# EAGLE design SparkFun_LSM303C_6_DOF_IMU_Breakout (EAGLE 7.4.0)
DESIGNER: Brent Wilkins; VERSION: v10
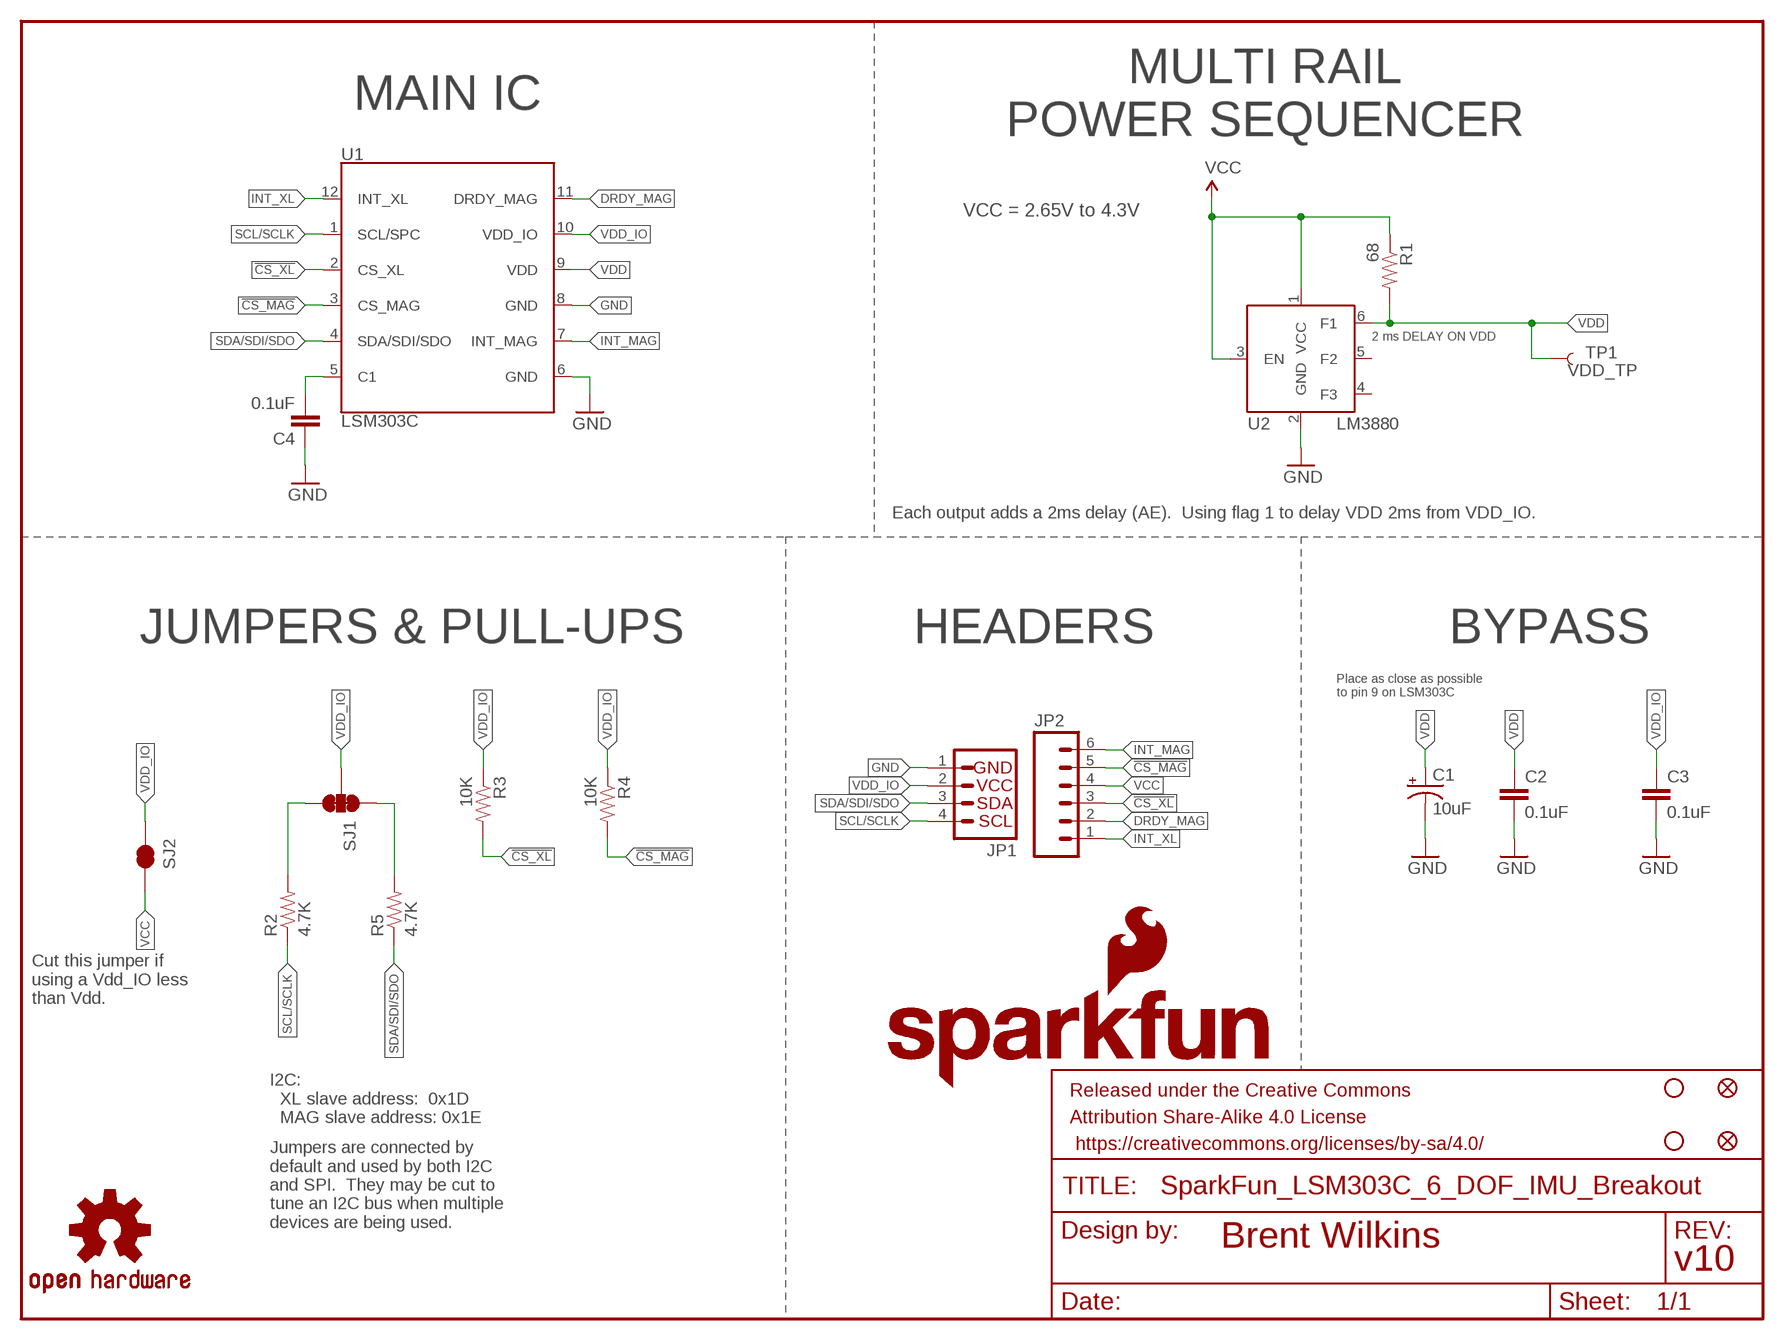
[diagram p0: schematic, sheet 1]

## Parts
C1  10uF  CAP_POL1206  [EIA3216]
C2  0.1uF  0.1UF-25V(+80/-20%)(0603)  [0603-CAP]
C3  0.1uF  0.1UF-25V(+80/-20%)(0603)  [0603-CAP]
C4  0.1uF  0.1UF-25V(+80/-20%)(0603)  [0603-CAP]
FID1  FIDUCIAL1X2  [FIDUCIAL-1X2]
FID2  FIDUCIAL1X2  [FIDUCIAL-1X2]
FRAME1  FRAME-LETTER  [CREATIVE_COMMONS]
JP1  I2C_STANDARD  [1X04]
JP2  M06SILK_FEMALE_PTH  [1X06]
LOGO1  SFE_LOGO_NAME.1_INCH  [SFE_LOGO_NAME_.1]
LOGO2  SFE_LOGO_FLAME.1EXP  [SFE_LOGO_FLAME_COPPER_EXPOSED_.1]
R1  68  RESISTOR0603-RES  [0603-RES]
R2  4.7K  4.7KOHM-1/10W-1%(0603)  [0603-RES]
R3  10K  10KOHM-1/10W-1%(0603)0603  [0603-RES]
R4  10K  10KOHM-1/10W-1%(0603)0603  [0603-RES]
R5  4.7K  4.7KOHM-1/10W-1%(0603)  [0603-RES]
SJ1  JUMPER-PAD-3-NC_BY_TRACE  [PAD-JUMPER-3-3OF3_NC_BY_TRACE_YES_SILK_FULL_BOX]
SJ2  JUMPER-PAD-2-NC_BY_TRACE  [PAD-JUMPER-2-NC_BY_TRACE_YES_SILK]
STANDOFF1  STAND-OFF  [STAND-OFF]
STANDOFF2  STAND-OFF  [STAND-OFF]
TP1  VDD_TP  TEST-POINTTP_15TH_THRU  [TP_15TH]
U1  LSM303C  [LGA-12]
U2  LM3880  LM3880/-QI  [SOT23-6]
U$8  OSHW-LOGOS  [OSHW-LOGO-S]

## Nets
!CS_MAG: JP2.5 R4.2 U1.3(CS_MAG)
!CS_XL: JP2.3 R3.2 U1.2(CS_XL)
DRDY_MAG: JP2.2 U1.11(DRDY_MAG)
GND: C1.C(-) C2.2 C3.2 C4.1 JP1.1 U1.6(GND) U1.8(GND) U2.2(GND)
I2C-UP: R5.2 SJ1.1
INT_MAG: JP2.6 U1.7(INT_MAG)
INT_XL: JP2.1 U1.12(INT_XL)
N$1: C4.2 U1.5(C1)
N$2: R2.2 SJ1.3
SCL/SCLK: JP1.4 R2.1 U1.1(SCL/SPC)
SDA/SDI/SDO: JP1.3 R5.1 U1.4(SDA/SDI/SDO)
VCC: JP2.4 R1.1 SJ2.2 U2.1(VCC) U2.3(EN)
VDD: C1.A(+) C2.1 R1.2 TP1.P$1 U1.9(VDD) U2.6(F1)
VDD_IO: C3.1 JP1.2 R3.1 R4.1 SJ1.2 SJ2.1 U1.10(VDD_IO)
Unconnected: U2.4(F3) U2.5(F2)

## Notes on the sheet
- MAIN IC
- MULTI RAIL
  POWER SEQUENCER
- VCC = 2.65V to 4.3V
- 2 ms DELAY ON VDD
- Each output adds a 2ms delay (AE).  Using flag 1 to delay VDD 2ms from VDD_IO.
- JUMPERS & PULL-UPS | HEADERS | BYPASS
- Place as close as possible
  to pin 9 on LSM303C
- Cut this jumper if
  using a Vdd_IO less
  than Vdd.
- I2C:
    XL slave address:  0x1D
    MAG slave address: 0x1E
- Jumpers are connected by
  default and used by both I2C
  and SPI.  They may be cut to
  tune an I2C bus when multiple
  devices are being used.

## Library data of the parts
C1 = SparkFun:CAP_POL: Capacitor Polarized; PROD_ID: CAP-00811
C2-C4 = SparkFun-Capacitors:0.1UF-25V(+80/-20%)(0603): CAP-00810; PROD_ID: CAP-00810
FID1 FID2 = SparkFun:FIDUCIAL: Fiducial Alignment Points
FRAME1 = SparkFun-Aesthetics:FRAME-LETTER: Schematic Frame
JP1 = SparkFun-Connectors:I2C_STANDARD: SparkFun has standardized on a pinout for all I2C based sensor breakouts. This pinout allows I2C boards to be plugged directly into the headers on Arduino Uno compatible boards, and to be daisy chained easily.
JP2 = SparkFun-Connectors:M06: Header 6 Standard 6-pin 0.1" header. Use with straight break away headers (SKU : PRT-00116), right angle break away headers (PRT-00553), swiss pins (PRT-00743), machine pins (PRT-00117), and female headers (PRT-00115). Molex polarized connector foot print use with SKU : PRT-08094 with associated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; PROD_ID: CONN-08437
LOGO1 = SparkFun-Aesthetics:SFE_LOGO_NAME: SFE Logo, name only
LOGO2 = SparkFun-Aesthetics:SFE_LOGO_FLAME: SFE Logo, flame only
R1 = SparkFun-Passives:RESISTOR: Resistor; PROD_ID: RES-07860
R2 R5 = SparkFun-Resistors:4.7KOHM-1/10W-1%(0603): RES-07857; PROD_ID: RES-07857
R3 R4 = SparkFun-Resistors:10KOHM-1/10W-1%(0603): RES-00824; PROD_ID: RES-00824
SJ1 = SparkFun-Passives:JUMPER-PAD-3-NC_BY_TRACE
SJ2 = SparkFun-Passives:JUMPER-PAD-2-NC_BY_TRACE
STANDOFF1 STANDOFF2 = SparkFun-Electromechanical:STAND-OFF: #4 Stand Off
TP1 = SparkFun-Passives:TEST-POINT: Bare copper test points for troubleshooting or ICT
U1 = SparkFun-DigitalIC:LSM303C: Ultra-compact high-performance eCompass module: 3D accelerometer and 3D magnetometer http://www.st.com/st-web-ui/static/active/en/resource/technical/document/datasheet/DM00089896.pdf; PROD_ID: IC-12557
U2 = SparkFun-DigitalIC:LM3880/-QI: Simple Power Sequencer Precision enable pin & 3 open-drain output flags Input Voltage Range of 2.7 V to 5.5 V Power-Up and Power-Down Control LM3880MF-1XY (Timing Designator) AF16ms AE2ms AA10ms AB30ms AC60ms AD120ms The timing sequence of the LM3880 is controlled entirely by the enable (EN) pin.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; PROD_ID: IC-12558
U$8 = SparkFun:OSHW-LOGO: Open Source Hardware Logo This logo indicates the piece of hardware it is found on incorporates a OSHW license and/or adheres to the definition of open source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

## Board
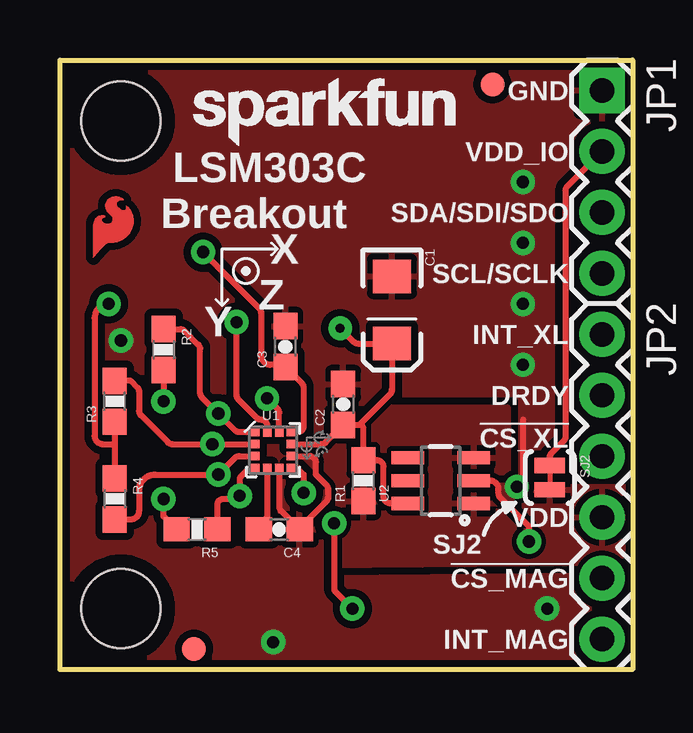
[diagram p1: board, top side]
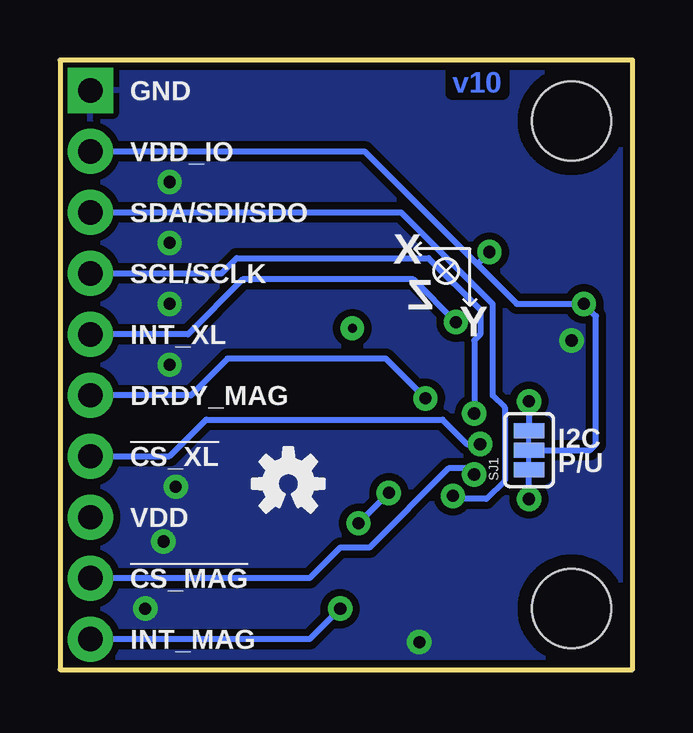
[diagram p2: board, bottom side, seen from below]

Size 23.88 x 25.4 mm. Coordinates in mm from the lower left corner, seen from the top.
Outline: 0,0 0,25.4 23.88,25.4 23.88,0 0,0
Copper layers (1*16): Top 0.035mm / dielectric 1.5mm / Bottom 0.035mm
Design rules "SparkFun-2-layer": minimum track width 7mil, minimum drill 15mil, track to track 8mil, track to pad 8mil, pad to pad 8mil, via to via 8mil, smd to smd 8mil, copper to edge 8mil, drill to drill 8mil, minimum pad ring 12mil, minimum via ring 10mil, stop-mask expansion 4mil, vias tented up to drill 20mil, thermal gap 10mil

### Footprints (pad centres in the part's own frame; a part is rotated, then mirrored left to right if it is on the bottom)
EIA3216 = smd 1.4 x 1.6: A 1.4,0; C -1.4,0
0603-CAP = smd 1.1 x 1: 1 -0.85,0; 2 0.85,0
FIDUCIAL-1X2 = smd 1 x 1: 1 0,0
1X04 = drill 1.016 pad 1.88 square: 1 0,0 | drill 1.016 pad 1.88: 2 2.54,0; 3 5.08,0; 4 7.62,0
1X06 = drill 1.016 pad 1.88: 1 0,0; 2 2.54,0; 3 5.08,0; 4 7.62,0; 5 10.16,0; 6 12.7,0
0603-RES = smd 1.1 x 1: 1 -0.85,0; 2 0.85,0
PAD-JUMPER-3-3OF3_NC_BY_TRACE_YES_SILK_FULL_BOX = smd 0.635 x 1.27: 1 -0.813,0; 2 0,0; 3 0.813,0
PAD-JUMPER-2-NC_BY_TRACE_YES_SILK = smd 0.635 x 1.27: 1 -0.508,0; 2 0.508,0
STAND-OFF = hole 3.302: 0,0
TP_15TH = drill 0.381 pad 0.61: P$1 0,0
LGA-12 = smd 0.375 x 0.35: 1 -0.75,0.75; 2 -0.75,0.25; 3 -0.75,-0.25; 4 -0.75,-0.75; 7 0.75,-0.75; 8 0.75,-0.25; 9 0.75,0.25; 10 0.75,0.75 | smd 0.35 x 0.375: 5 -0.25,-0.75; 6 0.25,-0.75; 11 0.25,0.75; 12 -0.25,0.75
SOT23-6 = smd 0.55 x 1.35: 1 -0.95,-1.375; 2 0,-1.375; 3 0.95,-1.375; 4 0.95,1.375; 5 0,1.375; 6 -0.95,1.375

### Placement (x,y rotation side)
C1  13.84,14.99 270 top
C2  11.81,11.05 90 top
C3  9.4,13.46 90 top
C4  9.14,5.84 180 top
FID1  18.03,24.38 0 top
FID2  5.59,0.86 0 top
FRAME1  not placed on the board
JP1  22.61,24.13 270 top
JP2  22.61,13.97 270 top
LOGO1  5.08,21.34 0 top
LOGO2  1.07,16.81 0 top
R1  12.65,7.87 90 top
R2  4.32,13.34 270 top
R3  2.29,11.18 90 top
R4  2.29,7.11 270 top
R5  5.71,5.84 180 top
SJ1  4.32,9.14 90 bottom
SJ2  20.42,8 270 top
STANDOFF1  2.54,22.86 0 top
STANDOFF2  2.54,2.54 0 top
TP1  11.68,14.22 0 top
U1  8.89,9.14 0 top
U2  15.88,7.87 90 top
U$8  14.35,7.75 0 bottom

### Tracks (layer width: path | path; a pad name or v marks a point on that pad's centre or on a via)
!CS_MAG  (via drill 0.51)
  Top 0.254: U1.3 7.47,8.89 arc45 7.3,8.82 v6.6,8.13 3.98,8.13 arc90 3.3,7.45 3.3,6.6 arc-90 2.96,6.26 R4.2
  Bottom 0.254: v6.6,8.13 6.86,8.38 7.67,8.38 10.97,5.08 12.19,5.08 13.46,3.81 JP2.5
!CS_XL  (via drill 0.51)
  Top 0.254: U1.2 v6.35,9.39 4.68,9.39 arc-45 4.5,9.47 3.38,10.59 arc-45 3.3,10.77 3.3,11.58 arc45 3.23,11.76 2.96,12.03 R3.2
  Bottom 0.254: JP2.3 19.3,8.89 17.78,10.41 7.92,10.41 6.91,9.4 v6.36,9.4 v6.35,9.39
DRDY_MAG  (via drill 0.51)
  Top 0.254: U1.11 9.14,10.69 arc45 9.07,10.87 v8.64,11.3
  Bottom 0.254: v8.64,11.3 10.29,12.95 16.89,12.95 18.41,11.43 JP2.2
GND  (via drill 0.51)
  Top 0.254: U1.6 9.14,6.8 arc45 9.22,6.62 C4.1 | U1.8 10.41,8.89 arc-90 10.67,8.64 10.67,8.13 11.1,7.69 arc-45 11.18,7.51 11.18,7.16 arc-45 11.11,7.01 10.03,5.93 arc45 C4.1 | 9.91,5.84 C4.1 | 19.3,10.41 19.3,7.87 v19.05,7.62 | v19.56,5.33 19.56,5.97 18.36,7.17 arc-45 18.29,7.34 18.29,7.52 arc90 17.93,7.87 U2.2
  other vias: 19.3,17.78 19.3,15.24 19.3,20.32 8.89,1.14 20.32,2.54 19.3,12.7 2.54,13.72
  pour Top (isolate 0.305, rank 6): 0,0 0,25.4 23.88,25.4 23.88,0
  pour Bottom (isolate 0.305): 0,0 0,25.4 23.88,25.4 23.88,0
I2C-UP  (via drill 0.51)
  Top 0.254: R5.2 4.32,6.39 v4.32,7.11
  Bottom 0.254: v4.32,7.11 SJ1.1
INT_MAG  (via drill 0.51)
  Top 0.254: U1.7 9.89,8.39 10.16,8.13 v10.16,7.37 | v11.43,6.1 11.43,3.41 arc45 11.5,3.23 v12.19,2.54
  Bottom 0.254: JP2.6 13.46,1.27 v12.19,2.54 | v10.16,7.37 v11.43,6.1
INT_XL  (via drill 0.51)
  Top 0.254: v7.37,14.48 7.37,11.43 arc45 7.44,11.25 8.21,10.49 arc45 8.39,10.41 arc-90 8.64,10.16 U1.12 8.64,10.16
  Bottom 0.254: JP2.1 18.54,13.97 16.26,16.26 9.14,16.26 v7.37,14.48
N$1
  Top 0.254: U1.5 8.64,6.35 8.29,6.01 C4.2 8.38,5.93
N$2  (via drill 0.51)
  Top 0.254: R2.2 v4.32,11.18
  Bottom 0.254: v4.32,11.18 SJ1.3
SCL/SCLK  (via drill 0.51)
  Top 0.254: R2.1 5.01,14.19 arc-45 5.19,14.11 5.77,13.54 arc-45 5.84,13.36 5.84,11.54 arc45 5.92,11.36 v6.6,10.67 7.3,9.97 arc45 7.48,9.89 U1.1
  Bottom 0.254: JP1.4 17.14,16.51 16.51,17.14 8.51,17.14 6.35,14.99 6.35,13.97 6.6,13.72 v6.6,10.67
SDA/SDI/SDO  (via drill 0.51)
  Top 0.254: U1.4 7.89,8.39 7.57,8.07 arc45 7.49,7.9 v7.49,7.24 7.37,7.11 6.81,7.11 arc90 6.57,6.87 R5.1
  Bottom 0.254: JP1.3 9.65,19.05 5.84,15.24 5.84,11.43 5.33,10.92 5.33,7.87 6.1,7.11 7.37,7.11 v7.49,7.24
VCC
  pour Top: 23.88,7.62 23.88,4.45 10.79,4.32 10.79,10.92 18.67,10.92 18.67,7.62
VDD
  Top 0.254: 12.48,10.2 C2.1 11.08,9.47 arc-45 10.9,9.39 U1.9 | 12.48,10.2 arc-90 12.65,10.04 R1.2 13.22,8.72 arc-45 13.4,8.65 13.41,8.63 arc-45 13.49,8.46 13.49,7.24 arc90 13.8,6.92 U2.6 | 12.48,10.2 13.77,11.48 arc45 13.84,11.66 C1.A 12.43,13.59 arc-45 12.25,13.66 TP1.P$1
VDD_IO  (via drill 0.51)
  Top 0.254: U1.10 9.65,9.91 9.91,9.91 9.89,9.89 U1.10 | R3.1 2.29,9.4 | 2.29,9.4 R4.1 | v2.03,15.24 arc90 1.45,14.66 1.45,9.73 arc90 1.78,9.4 2.29,9.4 | 9.4,12.7 8.74,12.7 arc-45 8.56,12.77 8.46,12.88 arc-45 8.38,13.06 8.38,14.88 arc45 8.31,15.06 v5.97,17.4 | JP1.2 21.16,20.14 arc45 21.08,19.96 21.08,9.71 arc-45 21.01,9.53 20.5,9.02 arc45 20.42,8.84 SJ2.1 | C3.1 10.09,11.92 arc-45 10.16,11.74 10.16,10.15 arc-90 9.91,9.89 U1.10
  Top 0.406: 9.4,12.7 C3.1
  Bottom 0.254: SJ1.2 1.78,9.14 1.52,9.4 1.52,14.73 v2.03,15.24 4.83,15.24 6.48,16.89 | JP1.2 11.18,21.59 6.48,16.89 | v5.97,17.4 6.48,16.89

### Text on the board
tPlace: GND | VDD_IO | SDA/SDI/SDO | LSM303C / Breakout | X | SCL/SCLK | Z | Y | INT_XL | DRDY | !CS_XL! | VDD | SJ2 | !CS_MAG | INT_MAG
bPlace: GND | VDD_IO | SDA/SDI/SDO | X | SCL/SCLK | Z | Y | INT_XL | DRDY_MAG | I2C | P/U | !CS_XL | VDD | !CS_MAG | INT_MAG
Measures: All units in inches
